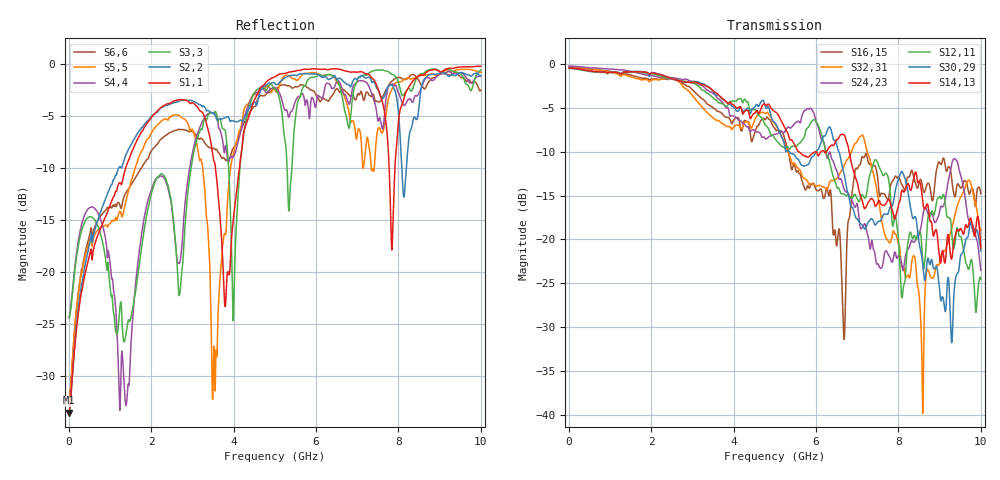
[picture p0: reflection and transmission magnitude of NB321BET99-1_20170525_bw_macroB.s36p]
! Touchstone(R) file created by SIwave 2017.0.0
! Touchstone(R) file created on Fri Jun 02 09:31:55 2017
! Port[1] = D_BN_0__DIE_409
! Port[2] = D_BN_0__LGA_B12
! Port[3] = D_BN_1__DIE_405
! Port[4] = D_BN_1__LGA_R31
! Port[5] = D_BN_2__DIE_401
! Port[6] = D_BN_2__LGA_A15
! Port[7] = D_BN_3__DIE_395
! Port[8] = D_BN_3__LGA_B16
! Port[9] = D_BN_4__DIE_385
! Port[10] = D_BN_4__LGA_A21
! Port[11] = D_BN_5__DIE_379
! Port[12] = D_BN_5__LGA_L31
! Port[13] = D_BN_6__DIE_375
! Port[14] = D_BN_6__LGA_J31
! Port[15] = D_BN_7__DIE_371
! Port[16] = D_BN_7__LGA_A23
! Port[17] = D_BP_0__DIE_408
! Port[18] = D_BP_0__LGA_A13
! Port[19] = D_BP_1__DIE_404
! Port[20] = D_BP_1__LGA_P30
! Port[21] = D_BP_2__DIE_400
! Port[22] = D_BP_2__LGA_B14
! Port[23] = D_BP_3__DIE_394
! Port[24] = D_BP_3__LGA_A17
! Port[25] = D_BP_4__DIE_384
! Port[26] = D_BP_4__LGA_B20
! Port[27] = D_BP_5__DIE_378
! Port[28] = D_BP_5__LGA_N31
! Port[29] = D_BP_6__DIE_374
! Port[30] = D_BP_6__LGA_G31
! Port[31] = D_BP_7__DIE_370
! Port[32] = D_BP_7__LGA_B22
! Port[33] = DCLK_BN_DIE_390
! Port[34] = DCLK_BN_LGA_B18
! Port[35] = DCLK_BP_DIE_389
! Port[36] = DCLK_BP_LGA_A19
! S-parameters (magnitude in dB)
# Hz S DB R 50.000000
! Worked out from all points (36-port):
!   1000 points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, 10 MHz to 10 GHz, reference 50 ohm
!   strongest paths, dB at 10 MHz, 2.51 GHz, 5.01 GHz, 7.51 GHz, 10 GHz:
!     S14,13: -0.4, -1.7, -5.4, -15.6, -21.0
!     S30,29: -0.4, -1.7, -6.7, -17.9, -21.3
!     S12,11: -0.5, -1.7, -8.5, -11.4, -24.5
!     S24,23: -0.2, -1.5, -8.0, -22.8, -23.5
!     S32,31: -0.3, -1.6, -6.8, -15.3, -18.9
!     S16,15: -0.3, -1.7, -7.4, -13.6, -14.8
!   lowest |S11| = -33.5 dB at 10 MHz (marker M1), VSWR 1.04, Z = 52.1 + j0.269 ohm
!   |S11| at or under -10 dB: start of sweep to 1.382 GHz; 3.561 GHz to 4.141 GHz (580.1 MHz wide, 15.1 % of centre); 7.774 GHz to 7.914 GHz (140 MHz wide, 1.78 % of centre)
